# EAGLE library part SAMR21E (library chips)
SAMR21E Cortex-M/802.15.4 SoC
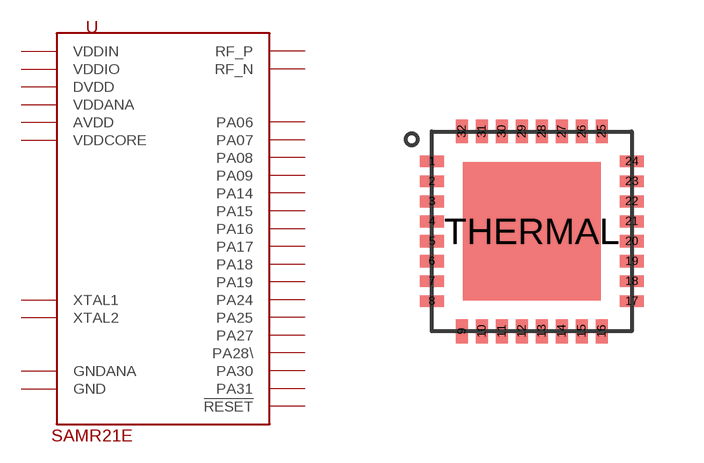
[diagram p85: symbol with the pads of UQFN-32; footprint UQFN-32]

Designator prefix U

## SAMR21E (DIGIKEY: 1611-ATSAMR21E18A-MUTCT-ND; MANUFACTURER: ATMEL; MPN: SAMR21E18A)  [UQFN-32]
1  XTAL2
2  XTAL1
3  GNDANA
4  VDDANA
5  AVDD
6  GNDANA
7  PA06
8  PA07
9  PA08
10  PA09
11  GNDANA
12  RF_P
13  RF_N
14  GNDANA
15  PA14
16  PA15
17  PA16
18  PA17
19  PA18
20  PA19
21  DVDD
22  PA24
23  PA25
24  VDDIO
25  PA27
26  !RESET
27  PA28\
28  GND
29  VDDCORE
30  VDDIN
31  PA30
32  PA31
THERMAL  GND

## Footprint UQFN-32 (pad centres in mm)
smd 0.6 x 0.3: 1 -2.5,1.75; 2 -2.5,1.25; 3 -2.5,0.75; 4 -2.5,0.25; 5 -2.5,-0.25; 6 -2.5,-0.75; 7 -2.5,-1.25; 8 -2.5,-1.75; 17 2.5,-1.75; 18 2.5,-1.25; 19 2.5,-0.75; 20 2.5,-0.25; 21 2.5,0.25; 22 2.5,0.75; 23 2.5,1.25; 24 2.5,1.75
smd 0.3 x 0.6: 9 -1.75,-2.5; 10 -1.25,-2.5; 11 -0.75,-2.5; 12 -0.25,-2.5; 13 0.25,-2.5; 14 0.75,-2.5; 15 1.25,-2.5; 16 1.75,-2.5; 25 1.75,2.5; 26 1.25,2.5; 27 0.75,2.5; 28 0.25,2.5; 29 -0.25,2.5; 30 -0.75,2.5; 31 -1.25,2.5; 32 -1.75,2.5
smd 3.45 x 3.45: THERMAL 0,0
